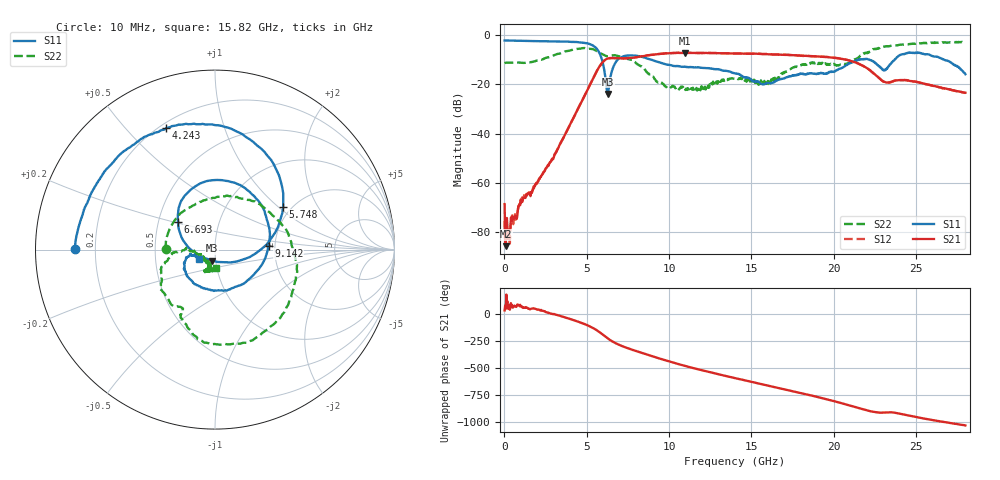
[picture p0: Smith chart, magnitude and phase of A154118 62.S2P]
!  2-Port S-parameters saved by WinCal
! VAR MeasName=S-Parameters (CALIBRATED_DATA) read from VNA (N5230A)
! VAR MeasDate=2015-9-10 14:39:53
! VAR NAME=A154118 62
! VAR FILENAME=A154118 62.S2P
! VAR DATE=2015-9-10 14:39:53
! VAR PHYS_PORTS=1,2
# Hz S DB R 50
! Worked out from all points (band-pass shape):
!   801 points, 10 MHz to 28 GHz, reference 50 ohm
!   highest |S21| = -7.18 dB at 10.96 GHz (marker M1); lowest = -85.7 dB at 79.97 MHz (marker M2)
!   |S21| within 3 dB of the highest: 6.086 GHz to 20.89 GHz (14.81 GHz wide, 110 % of centre)
!   lowest |S11| = -23.9 dB at 6.273 GHz (marker M3), VSWR 1.14, Z = 48.1 - j5.96 ohm
!   |S11| at or under -10 dB: 8.952 GHz to 21.45 GHz (12.5 GHz wide, 82.2 % of centre); 22.18 GHz to 23.69 GHz (1.518 GHz wide, 6.62 % of centre); 26.72 GHz to end of sweep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
!   |S22| runs from -22.8 to -2.7 dB; largest |S21 - S12| = 0.0082
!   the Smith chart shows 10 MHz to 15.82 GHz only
!   S11 on the Smith chart (normalised r, x): 10 MHz: 0.12, +0.00; 4.243 GHz: 0.23, +0.65; 5.748 GHz: 1.81, +1.08; 6.693 GHz: 0.63, +0.21; 9.142 GHz: 1.85, +0.08; 15.82 GHz: 0.83, -0.08
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1e7  -2.15 179.7  -68.60 32.2  -75.46 -58.0  -11.36 179.7
7.9975e7  -2.15 178.7  -85.68 45.9  -77.31 142.4  -11.19 176.1
3.248875e8  -2.20 175.2  -79.27 38.8  -85.36 61.2  -11.15 163.1
1.024638e9  -2.34 166.2  -67.99 72.0  -67.86 68.4  -11.21 126.6
2.38915e9  -2.46 147.9  -55.60 26.3  -55.46 24.9  -9.58 56.4
4.243488e9  -2.74 111.9  -32.94 -60.4  -32.98 -60.6  -5.72 -40.7
4.698325e9  -3.03 98.3  -26.87 -85.1  -26.87 -85.7  -5.35 -64.0
5.74795e9  -6.96 32.2  -12.98 -166.8  -13.00 -166.9  -7.10 -113.2
6.272762e9  -23.92 -104.3  -9.50 132.0  -9.47 132.0  -8.56 -119.9
6.692612e9  -11.79 143.1  -9.31 92.1  -9.31 92.0  -8.15 -128.2
7.70725e9  -8.23 81.0  -9.25 29.1  -9.26 29.0  -10.02 -161.7
9.141738e9  -10.49 3.9  -7.84 -41.9  -7.80 -42.0  -17.91 -176.6
9.351662e9  -10.91 -8.9  -7.69 -51.9  -7.64 -51.9  -19.03 -178.1
1.096109e10  -12.83 -92.2  -7.18 -123.0  -7.14 -123.5  -21.68 -134.7
1.239558e10  -13.42 -136.8  -7.23 -179.0  -7.19 -179.4  -20.76 -105.8
1.4005e10  -15.52 -163.3  -7.48 123.2  -7.47 122.6  -17.65 -113.7
1.582435e10  -19.72 -151.1  -7.66 59.8  -7.65 59.4  -19.58 -86.7
1.869332e10  -15.47 -134.9  -8.51 -40.3  -8.55 -40.9  -11.01 -90.1
2.117744e10  -10.90 -125.2  -10.74 -140.0  -10.79 -141.0  -9.91 -77.9
2.334666e10  -12.62 -128.7  -19.21 165.4  -19.23 164.3  -4.51 -98.8
2.516601e10  -7.13 -167.5  -19.18 116.9  -19.20 116.0  -3.40 -119.1
2.8e10  -15.84 137.7  -23.38 43.3  -23.48 43.2  -2.66 -141.1
